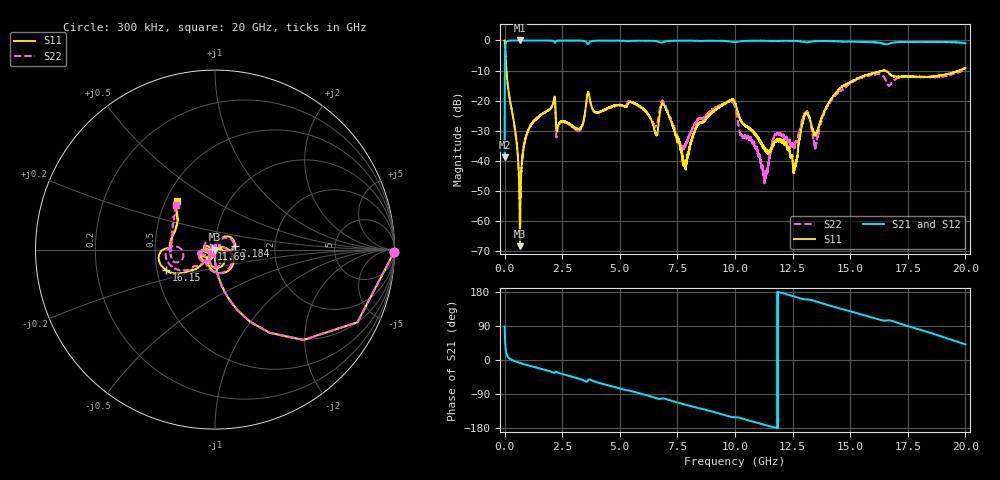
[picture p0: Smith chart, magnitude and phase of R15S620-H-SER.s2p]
!{R15S620}
!Johanson Technology Inc.
!www.johansontechnology.com
!Test Board Conditions:
!Substrate Type  RO4350B
!Substrate Thickness  20 mil
!Substrate Dk  3.66
!TL Type: GCPW
!TL Trace Width  34 mil
!TL Gap  10 mil
!Electrode orientation  Horizontal
!DUT TOPOLOGY	SERIES
!Mounting Pad LxW  26x52 mil
! Created Sat Feb  6 14:33:57 2021
# hz S ma R 50
! 2 Port Network Data from SP1.SP block
! freq  magS11  angS11  magS21  angS21  magS12  angS12  magS22  angS22
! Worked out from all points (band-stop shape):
!   20001 points, 300 kHz to 20 GHz, reference 50 ohm
!   highest |S21| = 0.00 dB at 651.3 MHz (marker M1); lowest = -38.8 dB at 300 kHz (marker M2)
!   |S21| within 3 dB of the highest: 26.28 MHz to end of sweep
!   lowest |S11| = -68.3 dB at 671.3 MHz (marker M3), VSWR 1.00, Z = 50 + j0.0196 ohm
!   |S11| at or under -10 dB: 77.51 MHz to 16.41 GHz (16.34 GHz wide, 198 % of centre); 16.41398 GHz to 16.4237 GHz (9.715 MHz wide, 0.0592 % of centre); 16.54 GHz to 19.71 GHz (3.171 GHz wide, 17.5 % of centre)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
!   |S22| runs from -67.9 to 0.0 dB; largest |S21 - S12| = 0.015
!   S11 on the Smith chart (normalised r, x): 300 kHz: open; 2.184 GHz: 1.24, +0.06; 11.69 GHz: 0.96, +0.01; 16.15 GHz: 0.56, -0.14; 20 GHz: 0.57, +0.35
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300000  0.9975 -0.9  0.01146 88.3  0.01149 88.9  0.9976 -0.8
1.143e8  0.2179 -78.5  0.9742 11.1  0.9752 11.1  0.2186 -78.7
6.513e8  0.002433 -88.8  1 -7.5  0.9989 -7.5  0.002024 -109.3
6.713e8  0.0003825 30.8  0.9987 -8.0  0.9991 -7.9  0.0006932 118.9
1.0903e9  0.0359 75.3  0.9983 -15.3  0.9986 -15.3  0.03714 76.1
2.1843e9  0.1113 11.7  0.9139 -33.0  0.9142 -33.0  0.1034 2.3
3.3343e9  0.03705 25.7  0.9914 -51.5  0.9912 -51.4  0.03497 28.6
3.6413e9  0.137 -74.1  0.8757 -52.0  0.8756 -52.0  0.1321 -81.8
6.6673e9  0.03638 -117.5  0.9553 -102.3  0.9551 -102.3  0.05128 -120.9
6.9293e9  0.08402 -160.8  0.952 -101.9  0.951 -101.9  0.0902 -164.4
7.8263e9  0.008004 91.6  0.991 -117.4  0.9918 -117.4  0.01767 -114.2
8.4083e9  0.04122 -19.6  0.9849 -127.0  0.984 -127.0  0.05035 -80.4
1.00003e10  0.09353 -101.7  0.9325 -150.8  0.9327 -150.8  0.07854 -112.7
1.13063e10  0.01478 -142.9  0.9867 -171.5  0.9883 -171.5  0.005644 28.9
1.16893e10  0.01962 166.3  0.9792 -177.5  0.9789 -177.5  0.02487 95.5
1.25963e10  0.008121 147.5  0.9805 167.1  0.9793 167.1  0.0181 137.0
1.30283e10  0.0579 -167.8  0.9343 160.1  0.9351 160.2  0.06417 163.6
1.33343e10  0.0365 156.2  0.9599 158.0  0.9592 157.9  0.03065 130.2
1.35053e10  0.02773 -169.2  0.9725 154.7  0.9728 154.8  0.01708 -175.9
1.61463e10  0.2954 -157.2  0.9263 108.7  0.9241 108.8  0.2759 -169.2
1.66673e10  0.2862 179.7  0.8778 104.7  0.8653 104.8  0.1788 -174.4
2e10  0.3463 128.0  0.9017 41.1  0.8954 40.9  0.3273 130.8
